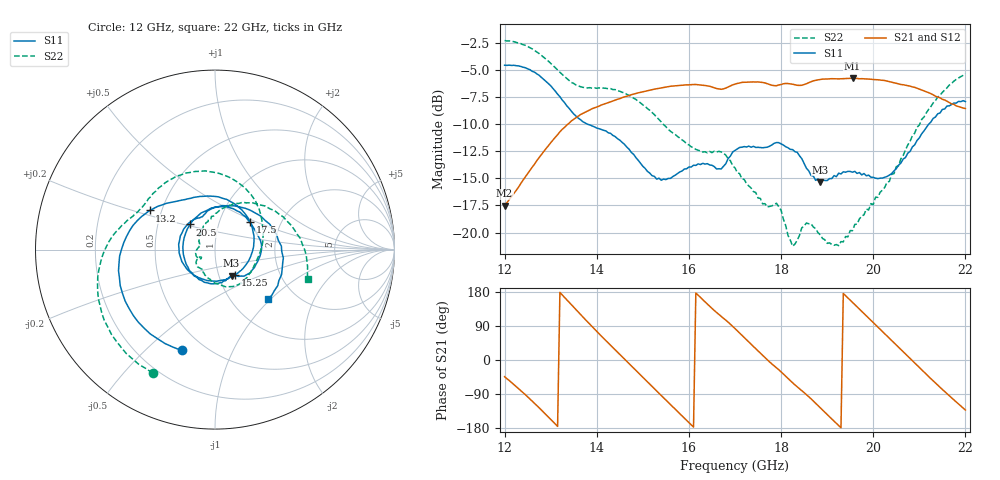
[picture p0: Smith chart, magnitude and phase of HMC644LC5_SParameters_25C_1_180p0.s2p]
!Analog Devices Inc..
!GaAs MMIC 5-BIT DIGITAL PHASE SHIFTER, 15 -8.5 GHz
!Filename: HMC644LC5_sparm_25C_1_0.s2p
!  :25C = 25degC
!  :_1_ = Sn1
!  :_180p0  = 180deg
!Device type:
!2 Port Calibration to sma connectors
!Phase Shifter:  0.000
!	50 Ohm System, Control Voltage = 0/-3V
!Freq	S11	S11	S21	S21	S12	S12	S22	S22
! GHz	Mag dB	Degrees	Mag dB	Degrees	Mag dB	Degrees	Mag dB	Degrees
# GHZ S DB R 50.0
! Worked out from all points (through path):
!   201 points, 12 GHz to 22 GHz, reference 50 ohm
!   highest |S21| = -5.75 dB at 19.55 GHz (marker M1); lowest = -17.5 dB at 12 GHz (marker M2)
!   lowest |S11| = -15.3 dB at 18.85 GHz (marker M3), VSWR 1.41, Z = 57.4 - j17.1 ohm
!   |S11| at or under -10 dB: 13.8 GHz to 21.2 GHz (7.402 GHz wide, 42.3 % of centre)
!   |S22| runs from -21.3 to -2.3 dB; largest |S21 - S12| = 0.0045
!   S11 on the Smith chart (normalised r, x): 12 GHz: 0.38, -0.65; 13.2 GHz: 0.43, +0.23; 15.25 GHz: 1.20, -0.35; 17.5 GHz: 1.40, +0.46; 20.5 GHz: 0.73, +0.21; 22 GHz: 1.45, -0.96
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12  -4.55 -108.4  -17.52 -44.0  -17.52 -44.0  -2.26 -116.8
12.55  -4.96 -159.2  -14.26 -102.9  -14.27 -102.7  -2.94 -154.0
13.2  -7.45 149.0  -10.70 178.4  -10.71 178.5  -5.20 168.1
13.7  -9.77 120.8  -8.99 113.4  -8.99 113.5  -6.59 148.7
14.1  -10.49 94.7  -8.22 63.0  -8.24 63.2  -6.68 130.1
14.55  -11.67 50.2  -7.54 8.3  -7.56 8.6  -7.05 100.9
15.25  -14.81 -51.6  -6.76 -75.8  -6.76 -75.7  -9.11 49.3
15.35  -14.98 -69.6  -6.67 -87.8  -6.66 -87.6  -9.56 42.2
16.15  -13.80 165.0  -6.33 177.0  -6.33 177.1  -12.32 -11.5
17  -12.42 86.5  -6.29 83.0  -6.29 83.0  -14.03 -82.8
17.5  -12.13 38.3  -6.09 23.9  -6.08 24.0  -16.81 -115.0
18.05  -11.92 -8.1  -6.26 -37.0  -6.25 -36.9  -18.77 -150.9
18.7  -14.79 -53.6  -5.99 -108.2  -5.99 -108.2  -19.49 -173.6
18.85  -15.33 -57.5  -5.86 -126.0  -5.85 -125.9  -20.21 176.3
19.2  -14.84 -74.5  -5.81 -167.1  -5.80 -167.0  -21.11 164.7
19.55  -14.43 -104.2  -5.75 152.1  -5.76 152.0  -19.83 149.9
19.95  -14.89 -145.9  -5.84 104.8  -5.83 105.0  -17.33 123.6
20.35  -14.70 158.8  -6.06 57.0  -6.05 57.2  -15.28 97.6
20.5  -14.10 134.8  -6.21 39.4  -6.21 39.3  -13.92 89.3
20.9  -11.90 73.6  -6.59 -7.9  -6.57 -7.7  -10.82 63.1
21.35  -9.33 18.9  -7.41 -60.6  -7.32 -60.6  -7.81 29.3
22  -7.90 -43.4  -8.55 -132.0  -8.64 -131.9  -5.34 -17.6
